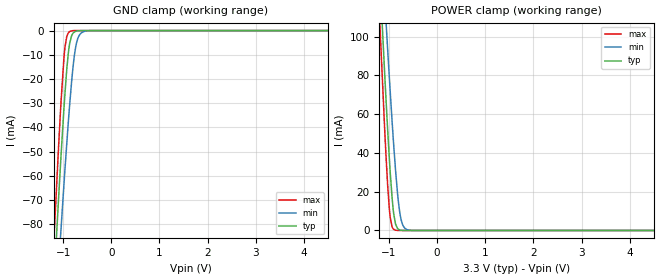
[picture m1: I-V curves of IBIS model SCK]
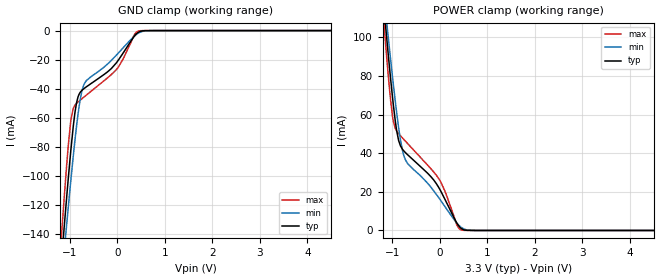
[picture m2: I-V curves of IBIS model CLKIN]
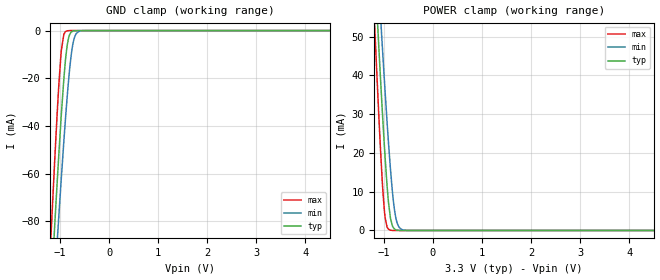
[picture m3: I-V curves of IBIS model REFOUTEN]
| Texas Instruments Incorporated
| 3-GHz, 8-Output Differential Fanout Buffer / Level Translator
| Marketing part#   Voltage Range   Package-type   #pins/pkg drawing
| LMK00308   3.15V - 3.45V   LLP   40-pin SQ
[IBIS Ver]   4.1
[File name]   lmk00308.ibs
[File Rev]   1.1
[Date]   1/29/2014
[Source]   Model built from spectre simulations at:
   Texas Instruments Incorporated.
   Analog-eLab, HPA
   12500 TI Blvd
   Dallas, TX -75243
   For Support e-mail: elab_ibis@list.ti.com
[Notes]   Revision History
   Rev 1.1: 01/28/2014
   - Add SCK buffer, update pin assignments
   Rev 1.0: 3/12/2012
   - ccomp values are based on PVT settings:
   WEAK: Low Voltage, High Temperature, Weak Process
   NOM: Nominal Voltage, Nominal Temperature, Nominal Process
   STRONG: High Voltage, Low Temperature, Fast Process
   - User may change ccomp in the order of number values as
   per end simulator used
   - C_comp although listed in numberical order of value are obtained from varying PVT conditions.
   For PVT conditions for eachspecific value, refer to the buffer description under repective [Model].
   IBIS model user is responsible for using appropriate C_comp to simulate for Signal Integrity.
   - LVPECL Simulation recommendation:
   Use low value (1nF or less) for AC coupling.
   Larger values will result in long settling times.
   -PullUp and Pulldown non-monotonic for LVPECL and REFOUT models
[Disclaimer]  This model is designed as an aid for customers of Texas Instruments
 TI and its licensors and suppliers make no warranties, either expressed
 or implied, with respect to this  model, including the warranties of
 merchantability or fitness for a particular purpose.
 The model is provided solely on an "as is" basis. The entire risk as to
 its quality and performance is with the customer.
[Copyright] (C)Copyright 2014 Texas Instruments Incorporated.
   All rights reserved.
[Component]   LMK00308SQ
[Manufacturer]  Texas Instruments Incorporated
[Package]   |40-pin LLP SQ package
|   typ   min   max
R_pkg   0   0   0
L_pkg   0   0   0
C_pkg   0   0   0
[Pin]   signal_name   model_name   R_pin   L_pin   C_pin
1   CLKoutA0   DIFFOUT
2   CLKoutA0*   DIFFOUT
3   VCC0A   POWER
4   CLKoutA1   DIFFOUT
5   CLKoutA1*   DIFFOUT
6   VCC0A   POWER
7   CLKoutA2   DIFFOUT
8   CLKoutA2*   DIFFOUT
9   CLKout32   DIFFOUT
10   CLKout32*   DIFFOUT
11   CLKoutA_TYPE0   SCK
12   VCC   POWER
13   OSCin   NC
14   OSCout   NC
15   CLKin_SEL0   SCK
16   CLKin0   CLKIN
17   CLKin0*   CLKIN
18   CLKin_SEL1   SCK
19   CLKoutB_TYPE0   SCK
20   GND   GND
21   CLKoutB3*   DIFFOUT
22   CLKoutB3   DIFFOUT
23   CLKoutB2*   DIFFOUT
24   CLKoutB2   DIFFOUT
25   VCC0B   POWER
26   CLKoutB1*   DIFFOUT
27   CLKoutB1   DIFFOUT
28   VCC0B   POWER
29   CLKoutB0*   DIFFOUT
30   CLKoutB0   DIFFOUT
31   GND   GND
32   CLKoutB_TYPE1   SCK
33   CLKin1*   CLKIN
34   CLKin1   CLKIN
35   VCC   POWER
36   REFout   REFOUT
37   VCC0C   POWER
38   REFout_EN   REFOUTEN
39   CLKoutA_TYPE1   SCK
40   GND   GND
41   DAP   NC
[Diff pin]  inv_pin  vdiff  tdelay_typ  tdelay_min  tdelay_max
 3   4   NA   0.0s   0.0s   0.0s
 6   7   NA   0.0s   0.0s   0.0s
 8   9   NA   0.0s   0.0s   0.0s
20   21   NA   0.0s   0.0s   0.0s
22   23   NA   0.0s   0.0s   0.0s
25   26   NA   0.0s   0.0s   0.0s
15   16   0.15   NA  NA  NA   | Diff-in
31   30   0.15   NA  NA  NA   | Diff-in
| Model REFOUT
[Model Selector]   REFOUT
REFOUT_33   3.3 volt Vcc
REFOUT_25   2.5 volt Vcc
| Model DIFFOUT
[Model Selector]   DIFFOUT
LVPECL_33   3.3 volt Vcc
LVPECL_25   2.5 volt Vcc
LVDS_33   3.3 volt Vcc
LVDS_25   2.5 volt Vcc
HCSL_33   3.3 volt Vcc
HCSL_25   2.5 volt Vcc
[Define Package Model]  llp40_lmk00308
[Manufacturer]  Unknown
[OEM]  Unknown
[Description]  ]  Evaled at 2GHz using Buildsheet AD#LMK00308SQ-01 RevA
[Number Of Pins]  41
[Pin Numbers]
|Pin Num   Terminal Name
1   | L1:1
2   | L2:2
3   | L3:3
4   | L4:4
5   | L5:5
6   | L6:6
7   | L7:7
8   | L8:8
9   | L9:9
10   | L10:10
11   | L11:11
12   | L12:12
13   | L13:13
14   | L14:14
15   | L15:15
16   | L16:16
17   | L17:17
18   | L18:18
19   | L19:19
20   | L20:20
21   | L21:21
22   | L22:22
23   | L23:23
24   | L24:24
25   | L25:25
26   | L26:26
27   | L27:27
28   | L28:28
29   | L29:29
30   | L30:30
31   | L31:31
32   | L32:32
33   | L33:33
34   | L34:34
35   | L35:35
36   | L36:36
37   | L37:37
38   | L38:38
39   | L39:39
40   | L40:40
41   | LDAP:41
[Model Data]
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[End Model Data]
[End Package Model]
| Models and submodels in the file (11): SCK (Input), CLKIN (Input), REFOUTEN (Input), LVPECL_25 (3-state), LVPECL_33 (3-state), LVDS_25 (Output), LVDS_33 (Output), HCSL_25 (Open_source), HCSL_33 (Open_source), REFOUT_25 (Output), REFOUT_33 (Output)
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|   Model SCK
[Model]   SCK
Model_type   Input
Vinl = 0.4
Vinh = 1.6
|   typ   min   max
|   (nom PVT)   (fast PVT)   (slow PVT)
C_comp   0.5966pF   0.57765pF   0.6104pF
[Voltage Range]   3.3   3.15   3.45
[Temperature Range]   27   125   -40
[Power Clamp Reference]   3.3   3.15   3.45
[GND Clamp Reference]   0   0   0
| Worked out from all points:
|   GND clamp passes 1 mA (typ) near -0.79 V on its own axis
|   POWER clamp passes 1 mA (typ) near -0.82 V on its own axis
[GND Clamp]
|   Voltage   I(typ)   I(min)   I(max)
-3.3V     -942.6mA   -854.7mA   -1.024A
-1.181V   -100.7mA   -125.5mA   -82.33mA
-1.092V   -68.4mA    -97.02mA   -46.97mA
-1.043V   -51.28mA   -81.58mA   -28.98mA
-963.6mV  -26.25mA   -57.73mA   -7.074mA
-924mV    -15.81mA   -46.4mA    -2.338mA
-864.6mV  -5.241mA   -30.59mA   -416.6uA
-785.4mV  -906.4uA   -13.39mA   -21.05uA
-726mV    -220.2uA   -5.463mA   -1.21uA
-656.7mV  -28.09uA   -1.707mA   0A
-537.9mV  -325.8nA   -217.8uA   0A
6.59V     0A         0A         0A
[POWER Clamp]
|   Voltage   I(typ)   I(min)   I(max)
-3.3V     1.303A     1.181A     1.417A
-1.191V   132mA      165.3mA    107.9mA
-1.181V   126.9mA    160.8mA    102.3mA
-1.092V   82.42mA    121.3mA    53.89mA
-1.063V   68.26mA    108.5mA    39.15mA
-993.3mV  37.62mA    79.36mA    11.46mA
-933.9mV  16.43mA    55.88mA    1.777mA
-864.6mV  3.384mA    31.47mA    134.7uA
-805.2mV  682.9uA    15.13mA    8.179uA
-745.8mV  107.4uA    5.402mA    0A
-577.5mV  0A         144uA      0A
6.59V     0A         0A         0A
|   Model   CLKIN
[Model]   CLKIN
Model_type   Input
Vinl = 1.2
Vinh = 1.35
|   typ   min   max
C_comp   0.334pF   0.334pF   0.334pF
[Voltage Range]   3.3   3.125   3.465
[Temperature Range]   45   125   -40
[Power Clamp Reference]   3.3   3.125   3.465
[GND Clamp Reference]   0   0   0
[GND Clamp]
|   Voltage   I(typ)   I(min)   I(max)
-3.3V     -1.09A     -1.005A    -1.209A
-1.181V   -161.9mA   -176mA     -145.1mA
-1.112V   -133.8mA   -150.7mA   -113.6mA
-1.063V   -114.4mA   -133.1mA   -92.33mA
-973.5mV  -81.6mA    -102.3mA   -61.43mA
-924mV    -65.73mA   -86.12mA   -53.42mA
-854.7mV  -49.53mA   -65.42mA   -49.97mA
-775.5mV  -42.3mA    -46.78mA   -47.7mA
-706.2mV  -40.03mA   -37.67mA   -45.84mA
-3.3mV    -21.51mA   -16.37mA   -26.2mA
432.3mV   -1.452mA   -2.001mA   -480.3uA
6.59V     0A         0A         0A
[POWER Clamp]
|   Voltage   I(typ)   I(min)   I(max)
-3.3V     736.4mA    674.5mA    821.9mA
-1.181V   117.5mA    123.8mA    109.8mA
-1.112V   98.9mA     107.1mA    88.87mA
-1.033V   78.62mA    88.59mA    67.5mA
-973.5mV  64.71mA    75.26mA    56.32mA
-914.1mV  53.13mA    62.75mA    51.87mA
-864.6mV  46.64mA    53.33mA    50.15mA
-745.8mV  40.96mA    38.12mA    46.9mA
-13.2mV   21.94mA    16.71mA    26.59mA
353.1mV   4.136mA    4.038mA    3.278mA
442.2mV   1.233mA    1.8mA      362.3uA
6.59V     0A         0A         0A
|   Model REFOUTEN
[Model]   REFOUTEN
Model_type   Input
Vinl = 0.8
Vinh = 2.0
|   typ   min   max
C_comp   0.3093pF   0.3093pF   0.3093pF
[Voltage Range]   3.3   3.125   3.465
[Temperature Range]   45   125   -40
[Power Clamp Reference]   3.3   3.125   3.465
[GND Clamp Reference]   0   0   0
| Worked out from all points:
|   GND clamp passes 1 mA (typ) near -0.79 V on its own axis
|   POWER clamp passes 1 mA (typ) near -0.82 V on its own axis
[GND Clamp]
|   Voltage   I(typ)   I(min)   I(max)
-3.3V     -965.6mA   -893.6mA   -1.069A
-1.181V   -108.3mA   -129.3mA   -84.35mA
-1.112V   -82.59mA   -106mA     -55.39mA
-1.043V   -57.82mA   -83.32mA   -28.72mA
-973.5mV  -34.81mA   -61.42mA   -8.124mA
-924mV    -20.4mA    -46.56mA   -1.597mA
-884.4mV  -11.09mA   -35.36mA   -347uA
-825mV    -2.889mA   -20.4mA    -26.1uA
-745.8mV  -310.8uA   -6.404mA   -528.4nA
-676.5mV  -33.31uA   -1.499mA   -14.52nA
-577.5mV  -943.1nA   -148.2uA   0A
6.59V     0A         0A         0A
[POWER Clamp]
|   Voltage   I(typ)   I(min)   I(max)
-3.3V     638.8mA    590.5mA    708.3mA
-1.191V   69.15mA    82.63mA    53.96mA
-1.181V   66.68mA    80.4mA     51.15mA
-1.102V   47.28mA    62.82mA    29.5mA
-1.033V   31.21mA    47.91mA    12.87mA
-993.3mV  22.67mA    39.68mA    5.73mA
-933.9mV  11.5mA     27.94mA    888.7uA
-864.6mV  3.112mA    15.73mA    67.37uA
-805.2mV  711.5uA    7.563mA    4.089uA
-745.8mV  145.3uA    2.701mA    212.4nA
-577.5mV  412.5nA    72uA       0A
6.59V     0A         0A         0A
